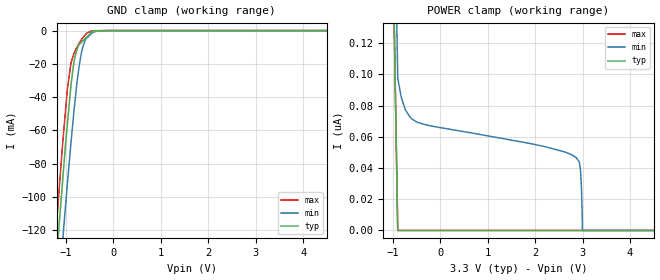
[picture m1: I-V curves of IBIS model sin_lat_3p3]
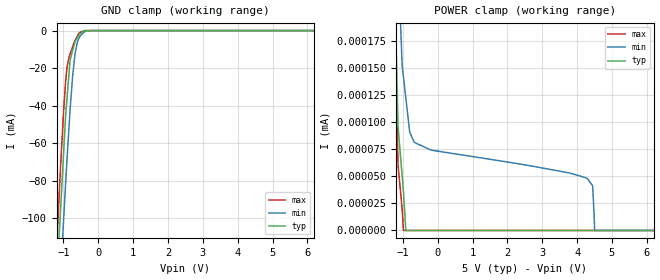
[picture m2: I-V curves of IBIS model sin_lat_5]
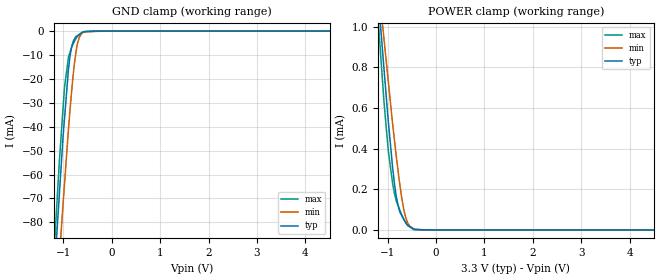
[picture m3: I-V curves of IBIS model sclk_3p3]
|Texas Instruments Incorporated
| 16 Channel Constant Current LED Driver with Pre-Charge FET
| Marketing part#   Digital Voltage Range   Package-type   #pins
| TLC59283DBQR   3.0V - 5.5V   SSOP   24
| TLC59283DBQ   3.0V - 5.5V   SSOP   24
| TLC59283DBQR   3.0V - 5.5V   QSOP   24
| TLC59283DBQ   3.0V - 5.5V   QSOP   24
| TLC59283RGER   3.0V - 5.5V   QFN   24
| TLC59283RGE   3.0V - 5.5V   QFN   24
[IBIS Ver]   3.2
[File name]   tlc59283.ibs
[File Rev]   1.0
[Date]   5/23/2012
[Source]
| Texas Instruments Incorporated.
| Analog-eLab Design Center, HPA
| 12500 TI Blvd
| Dallas, TX -75243
| e-mail: elab_scm_ibis@list.ti.com
[Notes]   Revision History:
| Rev 1.0: 5/23/2012
| - Initial version of the model
| - Model generated from simulations in TISPICE
| - Model matched to SPICE simulation
| - C_comp although listed in numerical order of value are
|   obtained from varying PVT conditions. For PVT conditions for
|   each specific value refer the buffer description under
|   respective [Model]. IBIS model user is responsible for using
|   appropriate C_comp to simulate for Signal Integrity.
| - Model names with a trailing _3p3 contains the model for
|   3.3V [3.0V and 3.6V]. Model names with a trailing _5 contains
|   the model for 5.0V [4.5V and 5.5V].
[Disclaimer]
| This model is designed as an aid for customers of Texas Instruments.
| TI and its licensors and suppliers make no warranties, either expressed
| or implied, with respect to this  model, including the warranties of
| merchantability or fitness for a particular purpose. The model is
| provided solely on an "as is" basis. The entire risk as to its quality
| and performance is with the customer.
[Copyright]
 (C) Copyright 2011 Texas Instruments Incorporated.All rights reserved.
|   TLC59283DBQ
[Component]   TLC59283DBQ
[Manufacturer]   TI
[Package]   |24 SSOP   -  DBQ package
|   typ   min   max
R_pkg   0.11729   0.08323   0.14535
L_pkg   3.22240nH   2.34736nH   4.63999nH
C_pkg   0.45953pF   0.38378pF   0.59375pF
[Pin]  signal_name   model_name   R_pin   L_pin   C_pin
1   GND   GND   0.05653   4.32900nH  0.70148pF
2   SIN   SIN_LAT   0.14531   4.15292nH  0.58579pF
3   SCLK   SCLK   0.13467   3.37419nH  0.44786pF
4   LAT   SIN_LAT   0.10850   2.81483nH  0.41275pF
5   OUT0   TERM   0.09164   2.50056nH  0.39387pF
6   OUT1   TERM   0.08323   2.34736nH  0.38378pF
7   OUT2   TERM   0.08587   2.39736nH  0.38695pF
8   OUT3   TERM   0.09850   2.63254nH  0.40102pF
9   OUT4   TERM   0.11725   2.98623nH  0.42167pF
10   OUT5   TERM   0.13914   3.46769nH  0.45276pF
11   OUT6   TERM   0.14343   4.12948nH  0.57603pF
12   OUT7   TERM   0.14265   4.63999nH  0.59375pF
13   OUT8   TERM   0.14265   4.63988nH  0.59374pF
14   OUT9   TERM   0.14342   4.12945nH  0.57605pF
15   OUT10   TERM   0.13914   3.46785nH  0.45274pF
16   OUT11   TERM   0.11725   2.98642nH  0.42163pF
17   OUT12   TERM   0.09850   2.63279nH  0.40099pF
18   OUT13   TERM   0.08587   2.39762nH  0.38698pF
19   OUT14   TERM   0.08323   2.34762nH  0.38390pF
20   OUT15   TERM   0.09164   2.50080nH  0.39389pF
21   BLANK   BLANK   0.10850   2.81488nH  0.41272pF
22   SOUT   SOUT   0.13467   3.37422nH  0.44778pF
23   IREF   TERM   0.14535   4.15817nH  0.58302pF
24   VCC   POWER   0.14247   4.63084nH  0.59537pF
|   TLC59283RGE
[Component]   TLC59283RGE
[Manufacturer]   TI
[Package]   |24 HTSSOP -  RGE package
|   typ   min   max
R_pkg   0.09171   0.08405   0.10271
L_pkg   1.55631nH   1.41448nH   1.75789nH
C_pkg   0.17849pF   0.14422pF   0.19672pF
[Pin]  signal_name   model_name   R_pin   L_pin   C_pin
1   LAT   SIN_LAT   0.09588   1.61052nH  0.16350pF
2   OUT0   TERM   0.08814   1.49739nH  0.18191pF
3   OUT1   TERM   0.08406   1.42337nH  0.17475pF
4   OUT2   TERM   0.08596   1.45690nH  0.17715pF
5   OUT3   TERM   0.09340   1.58991nH  0.18741pF
6   OUT4   TERM   0.10271   1.75789nH  0.19552pF
7   OUT5   TERM   0.10165   1.73808nH  0.19672pF
8   OUT6   TERM   0.08660   1.46709nH  0.17894pF
9   OUT7   TERM   0.08405   1.42472nH  0.14423pF
10   OUT8   TERM   0.08405   1.42382nH  0.14422pF
11   OUT9   TERM   0.08660   1.46429nH  0.17886pF
12   OUT10   TERM   0.10165   1.73317nH  0.19660pF
13   OUT11   TERM   0.10271   1.75050nH  0.19533pF
14   OUT12   TERM   0.09340   1.58201nH  0.18722pF
15   OUT13   TERM   0.08596   1.44819nH  0.17700pF
16   OUT14   TERM   0.08406   1.41448nH  0.17450pF
17   OUT15   TERM   0.08814   1.48899nH  0.18160pF
18   BLANK   BLANK   0.09588   1.63272nH  0.16321pF
19   SOUT   SOUT   0.09745   1.66222nH  0.16625pF
20   IREF   TERM   0.08886   1.50429nH  0.18433pF
21   VCC   POWER   0.08396   1.41687nH  0.17711pF
22   GND   GND   0.03144   1.12512nH  0.26658pF
23   SIN   SIN_LAT   0.08886   1.50631nH  0.18534pF
24   SCLK   SCLK   0.09745   1.66189nH  0.19228pF
|   Model Selectors
[Model Selector] SIN_LAT
sin_lat_3p3   3.3V digital input
sin_lat_5   5.0V digital input
[Model Selector] SCLK
sclk_3p3   3.3V digital input
sclk_5   5.0V digital input
[Model Selector] BLANK
blank_3p3   3.3V digital input
blank_5   5.0V digital input
[Model Selector] SOUT
sout_3p3   3.3V digital output
sout_5   5.0V digital output
[Model Selector] TERM
term_3-3V   3.3V nominal termination
term_5-0V   5.0V nominal termination
[Model] term_3-3V
Model_type Terminator
C_comp   1.0e-20F  1.0e-20F  1.0e-20F
|   typ   min   max
[Voltage Range]   3.3V   3.0V   3.6V
[POWER Clamp Reference]   3.3V   3.0V   3.6V
[GND Clamp Reference]   0V   0V   0V
|Ambient Temperature   25   85   -40
|Junction Temperature
[Temperature Range]   27   125   -40
[Model] term_5-0V
Model_type Terminator
C_comp   1.0e-20F  1.0e-20F  1.0e-20F
|   typ   min   max
[Voltage Range]   5.0V   4.5V   5.5V
[POWER Clamp Reference]   5.0V   4.5V   5.5V
[GND Clamp Reference]   0V   0V   0V
|Ambient Temperature   25   85   -40
|Junction Temperature
[Temperature Range]   27   125   -40
| Models and submodels in the file (10): sin_lat_3p3 (Input), sin_lat_5 (Input), sclk_3p3 (Input), sclk_5 (Input), blank_3p3 (Input), blank_5 (Input), sout_3p3 (Output), sout_5 (Output), term_3-3V (Terminator), term_5-0V (Terminator)
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|   sin_lat_3p3 Model
[Model]   sin_lat_3p3
Model_type   Input
Vinl = 0.99
Vinh = 2.31
|   typ   min   max
C_comp   1.569e-12   1.508e-12   1.693e-12
[Voltage Range]   3.3   3   3.6
|Ambient Temperature   25   85   -40
|Junction Temperature
[Temperature Range]   27   125   -40
[Power Clamp Reference]   3.3   3   3.6
[GND Clamp Reference]   0   0   0
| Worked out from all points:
|   GND clamp passes 1 mA (typ) near -0.46 V on its own axis
[GND Clamp]
|   Voltage   I(typ)   I(min)   I(max)
-3.3V     -999.5mA   -996.8mA   -1.011A
-1.256V   -158.6mA   -193.3mA   -138.4mA
-1.206V   -139.4mA   -174.7mA   -118.6mA
-1.165V   -123.7mA   -160mA     -103.1mA
-1.076V   -92.07mA   -128.3mA   -69.74mA
-1.032V   -76.2mA    -112.8mA   -55.16mA
-972mV    -56.46mA   -92.41mA   -35.46mA
-896.4mV  -33.25mA   -67.75mA   -19.59mA
-821.7mV  -17.43mA   -45.33mA   -13.01mA
-672mV    -6.956mA   -12.92mA   -5.342mA
-453.6mV  -749.8uA   -1.608mA   -114.4uA
6.6V      0A         0A         0A
[POWER Clamp]
|   Voltage   I(typ)   I(min)   I(max)
-3.3V     55.85uA    44.07uA    72.09uA
-1.365V   837.4nA    872nA      825.2nA
-897.6mV  0A         98.46nA    0A
-825mV    0A         85.44nA    0A
-741mV    0A         77.51nA    0A
-489mV    0A         69.33nA    0A
2.862V    0A         46.71nA    0A
2.928V    0A         43.92nA    0A
2.955V    0A         38.88nA    0A
2.979V    0A         23.94nA    0A
2.997V    0A         0A         0A
6.6V      0A         0A         0A
|   sin_lat_5 Model
[Model]   sin_lat_5
Model_type   Input
Vinl = 1.5
Vinh = 3.5
|   typ   min   max
C_comp   1.538e-12   1.458e-12   1.676e-12
| Where nom  PVT is Nominal Process, 5V, 27C
|   Fast PVT is Strong Process,  5.5V, -40C
|   Slow PVT is Weak Process,   4.5V, 125C
[Voltage Range]   5   4.5   5.5
|Ambient Temperature   25   85   -40
|Junction Temperature
[Temperature Range]   27   125   -40
[Power Clamp Reference]   5   4.5   5.5
[GND Clamp Reference]   0   0   0
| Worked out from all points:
|   GND clamp passes 1 mA (typ) near -0.48 V on its own axis
[GND Clamp]
|   Voltage   I(typ)   I(min)   I(max)
-5V       -1.725A    -1.694A    -1.759A
-1.188V   -132.8mA   -168.2mA   -111.6mA
-1.14V    -114.5mA   -151mA     -93.53mA
-1.089V   -97mA      -132.8mA   -74.3mA
-1.026V   -75.37mA   -110.8mA   -52.62mA
-1.001V   -66.78mA   -102.3mA   -44.07mA
-929.5mV  -42.88mA   -78.4mA    -25.19mA
-810mV    -15.72mA   -42.02mA   -12.44mA
-675mV    -6.197mA   -13.33mA   -5.563mA
-544.5mV  -2.036mA   -3.503mA   -1.115mA
-396mV    -247.9uA   -578uA     -17.49uA
10V       0A         0A         0A
[POWER Clamp]
|   Voltage   I(typ)   I(min)   I(max)
-5V       89.11uA    69.65uA    115.2uA
-1.232V   240nA      423.2nA    187.8nA
-1.215V   199nA      383.7nA    164.6nA
-1.139V   95.83nA    255.1nA    60.2nA
-984.5mV  36.41nA    142.1nA    0A
-915mV    0A         122.4nA    0A
-805.5mV  0A         91.34nA    0A
-670.5mV  0A         81.42nA    0A
4.253V    0A         48.73nA    0A
4.446V    0A         41.29nA    0A
4.505V    0A         0A         0A
10V       0A         0A         0A
|   sclk_3p3 Model
[Model]   sclk_3p3
Model_type   Input
Vinl = 0.99
Vinh = 2.31
|   typ   min   max
C_comp   5.648e-13   5.404e-13   5.892e-13
| Where nom  PVT is Nominal Process, 3.3V, 27C
|   Fast PVT is Strong Process,  3.6V, -40C
|   Slow PVT is Weak Process,   3V, 125C
[Voltage Range]   3.3   3   3.6
|Ambient Temperature   25   85   -40
|Junction Temperature
[Temperature Range]   27   125   -40
[Power Clamp Reference]   3.3   3   3.6
[GND Clamp Reference]   0   0   0
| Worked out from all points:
|   GND clamp passes 1 mA (typ) near -0.64 V on its own axis
|   POWER clamp passes 1 mA (typ) near -1.15 V on its own axis
[GND Clamp]
|   Voltage   I(typ)   I(min)   I(max)
-3.3V     -909.7mA   -876.9mA   -959mA
-1.171V   -95.35mA   -122mA     -84.37mA
-1.087V   -68.76mA   -95.9mA    -55.07mA
-1.032V   -51.35mA   -78.82mA   -38.92mA
-979.2mV  -36.62mA   -63.98mA   -23.48mA
-896.4mV  -15.79mA   -40.74mA   -10.8mA
-864.6mV  -10.36mA   -32.83mA   -8.854mA
-807mV    -4.874mA   -19.75mA   -5.678mA
-732mV    -2.18mA    -7.467mA   -2.824mA
-672mV    -1.384mA   -2.584mA   -1.489mA
-590.7mV  -305.7uA   -561.6uA   -382.9uA
6.6V      0A         0A         0A
[POWER Clamp]
|   Voltage   I(typ)   I(min)   I(max)
-3.3V     8.146mA    6.63mA     9.069mA
-1.213V   1.208mA    1.258mA    1.087mA
-1.142V   984.9uA    1.091mA    848.6uA
-1.076V   792.5uA    938.3uA    630.4uA
-986.4mV  532.1uA    728.1uA    386.6uA
-897.6mV  305.3uA    520.7uA    228.1uA
-821.7mV  164.8uA    360.7uA    142.5uA
-714mV    72.64uA    164.5uA    76.74uA
-627mV    33.96uA    60.96uA    38.39uA
-534mV    15.01uA    16.71uA    13.38uA
-453.6mV  2.741uA    5.423uA    1.489uA
6.6V      0A         0A         0A
